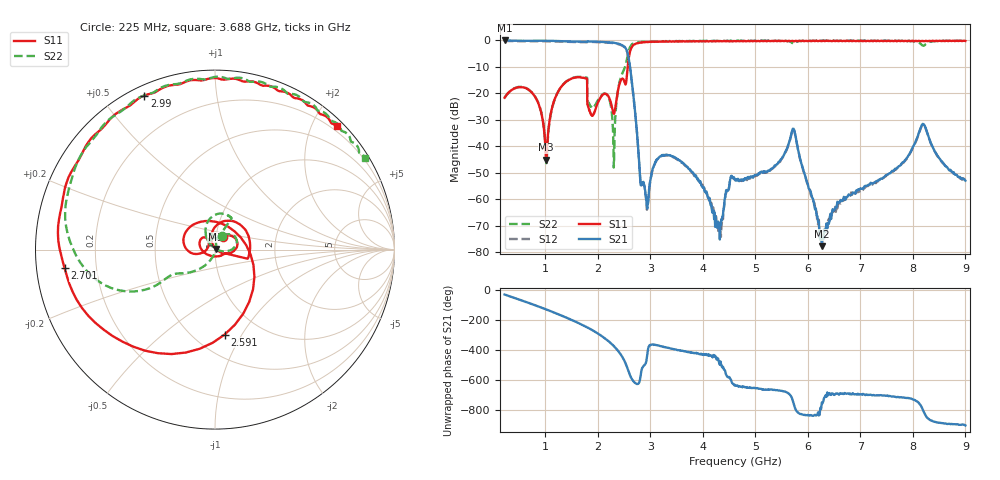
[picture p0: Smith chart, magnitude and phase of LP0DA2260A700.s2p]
!Agilent Technologies,E8358A,US41080443,A.07.50.56
!Agilent E8358A: A.07.50.56
!Date: Monday, May 09, 2016 11:37:28
!Correction: S11(Full 2 Port(1,2))
!S21(Full 2 Port(1,2))
!S12(Full 2 Port(1,2))
!S22(Full 2 Port(1,2))
!S2P File: Measurements: S11, S21, S12, S22:Log Frequency Sweep
# Hz S  dB  R 50
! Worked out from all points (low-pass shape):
!   1601 points, 225 MHz to 9 GHz, reference 50 ohm
!   highest |S21| = 0.00 dB at 226.6 MHz (marker M1); lowest = -77.8 dB at 6.267 GHz (marker M2)
!   |S21| within 3 dB of the highest: start of sweep to 2.533 GHz
!   lowest |S11| = -45.1 dB at 1.019 GHz (marker M3), VSWR 1.01, Z = 50.4 + j0.417 ohm
!   |S11| at or under -10 dB: start of sweep to 2.569 GHz
!   |S22| runs from -48.1 to 0.0 dB; largest |S21 - S12| = 0.021
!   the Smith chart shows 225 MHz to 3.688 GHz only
!   S11 on the Smith chart (normalised r, x): 225 MHz: 1.08, +0.15; 2.591 GHz: 0.69, -0.85; 2.701 GHz: 0.08, -0.06; 2.99 GHz: 0.04, +0.64; 3.688 GHz: 0.11, +2.39
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2.25e8  -21.66 59.1  -0.01 -27.8  -0.17 -27.6  -21.59 61.7
2.265616e8  -21.60 58.9  -0.00 -28.0  -0.17 -27.8  -21.52 61.6
7.868313e8  -20.73 -10.5  -0.12 -96.6  -0.29 -96.5  -20.64 -0.1
1.018652e9  -45.14 48.4  -0.12 -127.2  -0.29 -127.1  -46.10 43.5
1.210939e9  -20.68 101.0  -0.19 -153.9  -0.36 -153.8  -20.68 122.9
1.687749e9  -14.03 14.3  -0.48 133.1  -0.64 133.1  -13.78 71.2
2.25668e9  -24.15 127.0  -0.77 5.2  -0.93 5.2  -25.77 86.3
2.457637e9  -14.53 157.2  -1.72 -78.6  -1.89 -78.4  -12.84 -144.7
2.591476e9  -6.43 -83.6  -7.15 173.7  -7.27 173.9  -3.76 -162.4
2.701285e9  -1.47 -173.0  -25.33 105.4  -25.46 105.7  -0.93 151.1
2.83529e9  -0.78 144.1  -54.67 -167.5  -54.82 -167.7  -0.53 119.8
2.989696e9  -0.49 114.7  -54.36 -7.3  -54.24 -4.8  -0.40 95.1
3.152512e9  -0.47 93.3  -44.57 -7.9  -44.51 -8.0  -0.33 76.5
3.687604e9  -0.29 45.3  -47.56 -48.8  -47.61 -48.2  -0.17 31.5
4.303586e9  -0.32 10.3  -70.41 -114.2  -70.97 -95.4  -0.21 -0.5
4.622431e9  -0.31 -2.9  -52.99 85.4  -52.53 85.6  -0.14 -12.2
5.71464e9  -0.18 -33.9  -33.38 -17.7  -33.61 -17.7  -1.14 -39.7
6.081681e9  -0.17 -40.8  -59.41 -115.4  -60.28 -111.4  -0.10 -42.2
6.266721e9  -0.24 -44.9  -77.80 -27.1  -74.81 -65.1  -0.10 -45.6
7.553438e9  -0.23 -73.4  -50.18 16.4  -50.28 13.3  -0.12 -70.6
8.188224e9  -0.17 -86.4  -31.54 -75.0  -31.73 -75.0  -1.94 -84.1
9e9  -0.19 -98.8  -53.01 179.4  -52.31 -177.1  -0.11 -96.7
